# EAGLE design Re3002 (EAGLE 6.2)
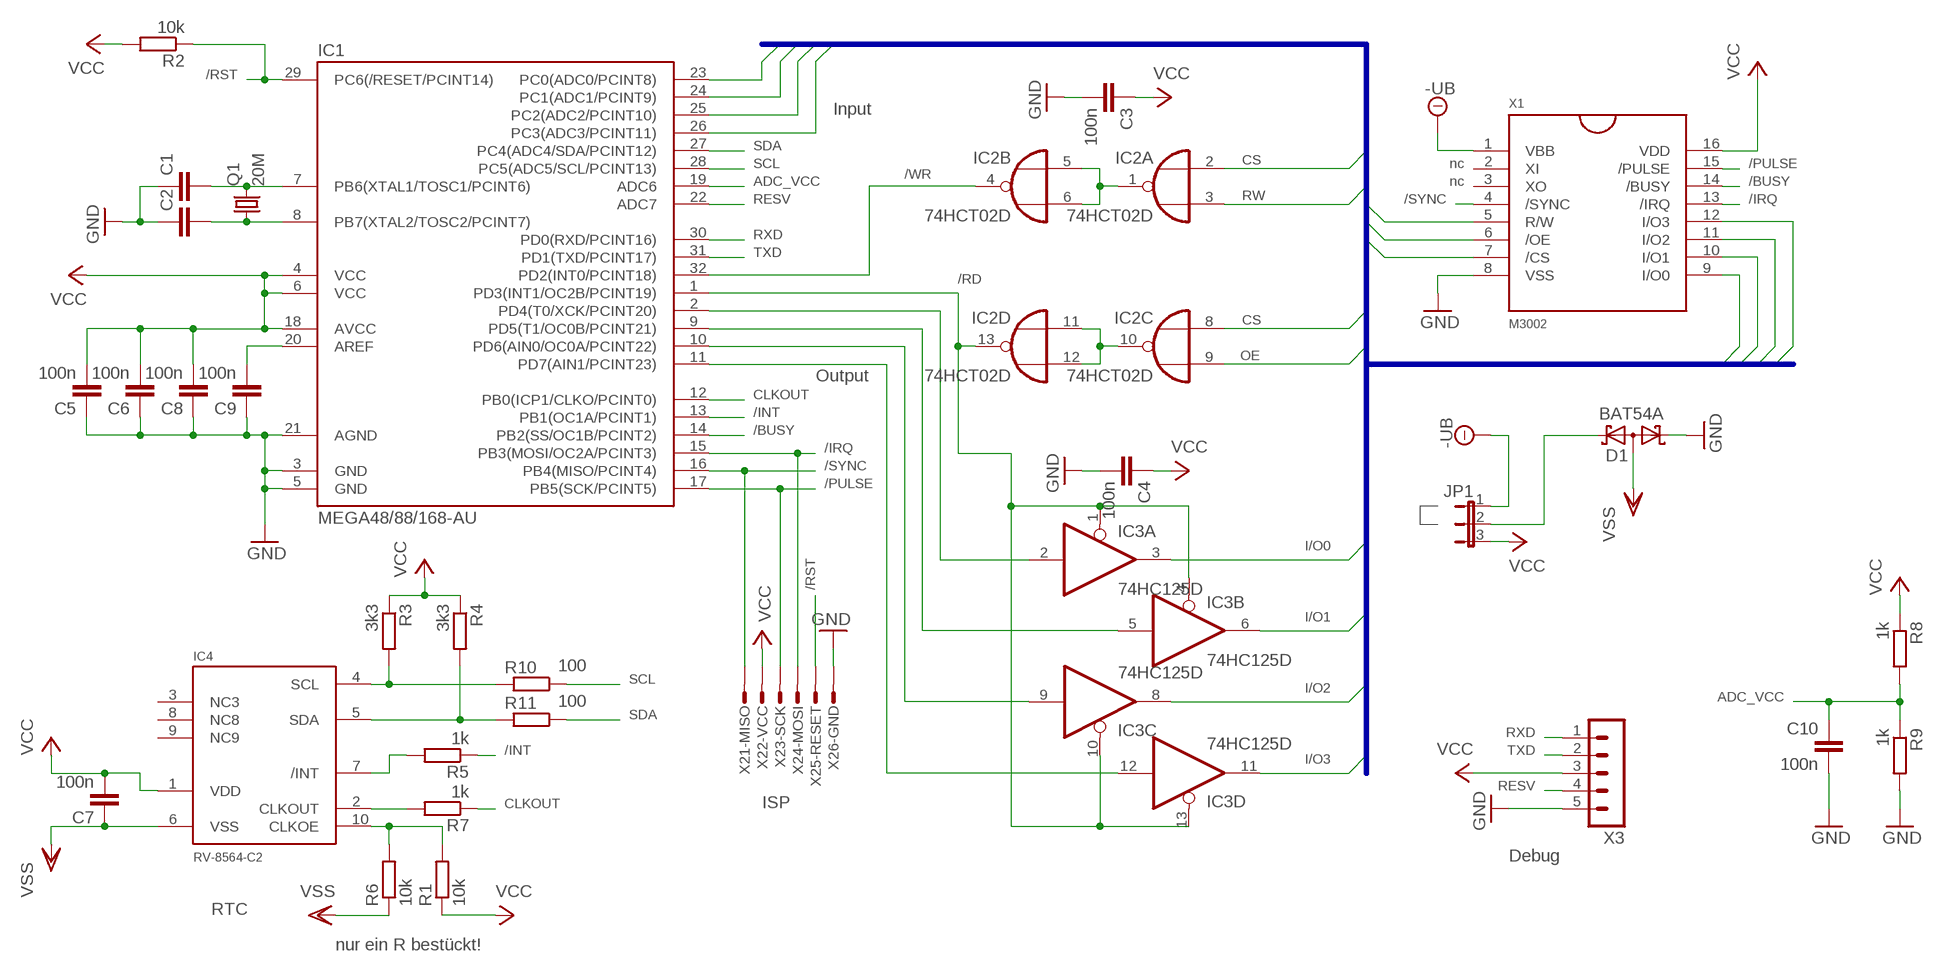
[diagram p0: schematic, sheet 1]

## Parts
C1  C-EUC0603  [C0603]
C2  C-EUC0603  [C0603]
C3  100n  C-EUC0603  [C0603]
C4  100n  C-EUC0603  [C0603]
C5  100n  C-EUC0603  [C0603]
C6  100n  C-EUC0603  [C0603]
C7  100n  C-EUC0603  [C0603]
C8  100n  C-EUC0603  [C0603]
C9  100n  C-EUC0603  [C0603]
C10  100n  C-EUC0603  [C0603]
D1  BAT54A  [SOT23]
IC1  MEGA48/88/168-AU  [TQFP32-08]
IC2  74HCT02D  [SO14]
IC3  74HC125D  [SO14]
IC4  RV-8564-C2  [RTC-MCS-50X32]
JP1  JP2E  [JP2]
Q1  20M  CRYSTALHC49S  [HC49/S]
R1  10k  R-EU_R0603  [R0603]
R2  10k  R-EU_R0603  [R0603]
R3  3k3  R-EU_R0603  [R0603]
R4  3k3  R-EU_R0603  [R0603]
R5  1k  R-EU_R0603  [R0603]
R6  10k  R-EU_R0603  [R0603]
R7  1k  R-EU_R0603  [R0603]
R8  1k  R-EU_R0603  [R0603]
R9  1k  R-EU_R0603  [R0603]
R10  100  R-EU_R0603  [R0603]
R11  100  R-EU_R0603  [R0603]
X1  M3002  [DIL-16]
X2  AVR-ISP_1X6  [1X6_ISP]
X3  MA05-1  [MA05-1]

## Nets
-UB: JP1.1 X1.1(VBB)
/BUSY: IC1.14(PB2(SS/OC1B/PCINT2)) X1.14(/BUSY)
/INT: IC1.13(PB1(OC1A/PCINT1)) R5.1
/IRQ: IC1.15(PB3(MOSI/OC2A/PCINT3)) X1.13(/IRQ) X2.4
/PULSE: IC1.17(PB5(SCK/PCINT5)) X1.15(/PULSE) X2.3
/RD: IC1.1(PD3(INT1/OC2B/PCINT19)) IC2.13(D:O) IC3.1(A:OE) IC3.4(B:OE) IC3.10(C:OE) IC3.13(D:OE)
/RST: IC1.29(PC6(/RESET/PCINT14)) R2.1 X2.5
/SYNC: IC1.16(PB4(MISO/PCINT4)) X1.4(/SYNC) X2.1
/WR: IC1.32(PD2(INT0/PCINT18)) IC2.4(B:O)
ADC_VCC: C10.1 IC1.19(ADC6) R8.2 R9.1
AREF: C9.2 IC1.20(AREF)
CLKOUT: IC1.12(PB0(ICP1/CLKO/PCINT0)) R7.1
CS: IC2.2(A:I0) IC2.8(C:I0) X1.7(/CS)
GND: C1.1 C2.1 C3.2 C4.2 C5.1 C6.1 C8.1 C9.1 C10.2 D1.1(K1) IC1.3(GND) IC1.5(GND) IC1.21(AGND) R9.2 X1.8(VSS) X2.6 X3.5
I/O0: IC1.23(PC0(ADC0/PCINT8)) IC3.3(A:O) X1.9(I/O0)
I/O1: IC1.24(PC1(ADC1/PCINT9)) IC3.6(B:O) X1.10(I/O1)
I/O2: IC1.25(PC2(ADC2/PCINT10)) IC3.8(C:O) X1.11(I/O2)
I/O3: IC1.26(PC3(ADC3/PCINT11)) IC3.11(D:O) X1.12(I/O3)
N$1: IC2.1(A:O) IC2.5(B:I0) IC2.6(B:I1)
N$2: IC2.10(C:O) IC2.11(D:I0) IC2.12(D:I1)
N$3: D1.2(K2) JP1.2
N$5: IC4.4(SCL) R3.2 R10.2
N$6: IC4.5(SDA) R4.2 R11.2
N$7: IC4.2(CLKOUT) R7.2
N$8: IC4.7(/INT) R5.2
N$9: C1.2 IC1.7(PB6(XTAL1/TOSC1/PCINT6)) Q1.2
N$10: C2.2 IC1.8(PB7(XTAL2/TOSC2/PCINT7)) Q1.1
N$12: IC4.10(CLKOE) R1.2 R6.2
OE: IC2.9(C:I1) X1.6(/OE)
OUT0: IC1.2(PD4(T0/XCK/PCINT20)) IC3.2(A:I)
OUT1: IC1.9(PD5(T1/OC0B/PCINT21)) IC3.5(B:I)
OUT2: IC1.10(PD6(AIN0/OC0A/PCINT22)) IC3.9(C:I)
OUT3: IC1.11(PD7(AIN1/PCINT23)) IC3.12(D:I)
RESV: IC1.22(ADC7) X3.4
RW: IC2.3(A:I1) X1.5(R/W)
RXD: IC1.30(PD0(RXD/PCINT16)) X3.1
SCL: IC1.28(PC5(ADC5/SCL/PCINT13)) R10.1
SDA: IC1.27(PC4(ADC4/SDA/PCINT12)) R11.1
TXD: IC1.31(PD1(TXD/PCINT17)) X3.2
VCC: C3.1 C4.1 C5.2 C6.2 C7.2 C8.2 IC1.4(VCC) IC1.6(VCC) IC1.18(AVCC) IC4.1(VDD) JP1.3 R1.1 R2.2 R3.1 R4.1 R8.1 X1.16(VDD) X2.2 X3.3
VSS: C7.1 D1.3(AA) IC4.6(VSS) R6.1
Unconnected: IC4.3(NC3) IC4.8(NC8) IC4.9(NC9) X1.2(XI) X1.3(XO)

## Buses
I/O[0..3],CS,RW,OE

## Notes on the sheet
- Input
- nc
- nc
- Output
- ISP
- Debug
- RTC
- nur ein R bestückt!

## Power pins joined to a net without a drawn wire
GND: IC2.7(P:GND) IC3.7(P:GND)
VCC: IC2.14(P:VCC) IC3.14(P:VCC)

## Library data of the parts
C1-C10 = rcl:C-EU: CAPACITOR, European symbol
D1 = diode:BAT54A: Schottky Diodes Source: Fairchild .. BAT54.pdf
IC1 = avr-7:MEGA48/88/168
IC2 = 74xx-eu:74*02: Quad 2-input NOR gate
IC3 = 74xx-eu:74*125: Quad bus BUFFER, 3-state
IC4 = misc:RV-8564-C2
JP1 = jumper:JP2E: JUMPER
Q1 = crystal:CRYSTAL: CRYSTAL; OC_FARNELL: 1667008; OC_NEWARK: unknown
R1-R11 = rcl:R-EU_: RESISTOR, European symbol
X1 = misc:M3002
X2 = 0_rr:AVR-ISP: MicroMaTch 6 7-215464-6 / 0-215464-6 Drawing Number C-215464 DDEController.pdf
X3 = con-lstb:MA05-1: PIN HEADER; OC_FARNELL: unknown; OC_NEWARK: unknown

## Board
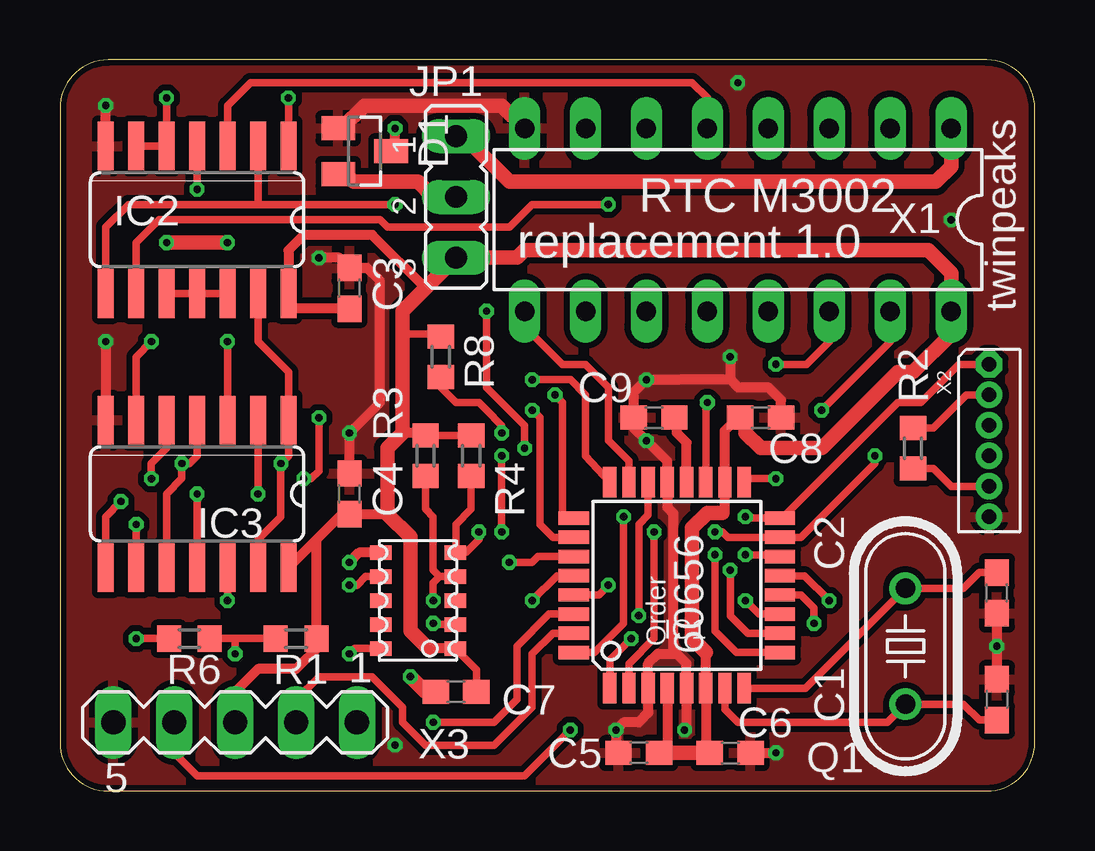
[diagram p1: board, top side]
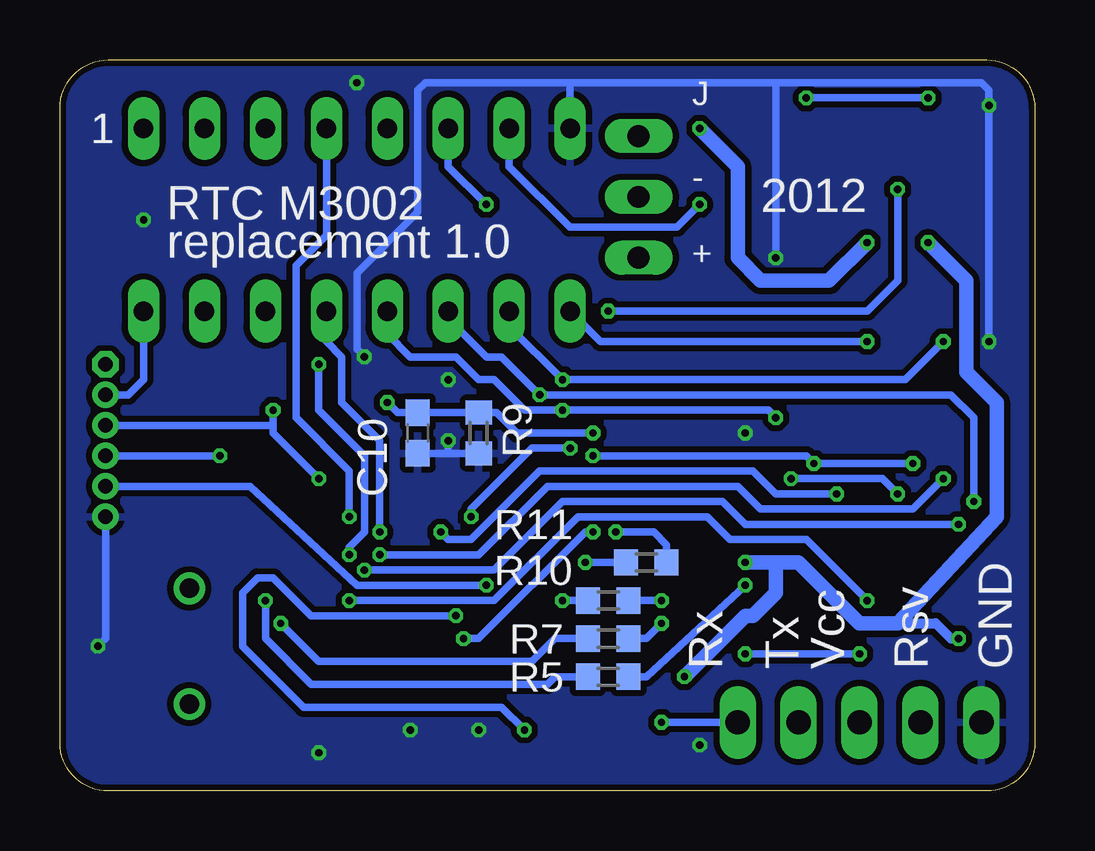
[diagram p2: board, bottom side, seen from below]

Size 40.63 x 30.47 mm. Coordinates in mm from the lower left corner, seen from the top.
Outline: 0,28.47 0,2 arc90 2,0 38.63,0 arc90 40.63,2 40.63,28.47 arc90 38.63,30.47 2,30.47 arc90 0,28.47
Copper layers (1*16): Top 0.035mm / dielectric 1.5mm / Bottom 0.035mm
Design rules: minimum track width 6mil, minimum drill 12mil, track to track 6mil, track to pad 6mil, pad to pad 6mil, via to via 6mil, smd to smd 0mil, copper to edge 10mil, drill to drill 10mil, minimum pad ring 10mil, minimum via ring 6mil, stop-mask expansion 2mil, vias tented up to drill 100mil, thermal gap 10mil

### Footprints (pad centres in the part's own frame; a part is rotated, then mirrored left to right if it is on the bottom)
C0603 = smd 1.1 x 1: 1 -0.85,0; 2 0.85,0
SOT23 = smd 1 x 1.4: 1 -0.95,-1.1; 2 0.95,-1.1; 3 0,1.1
TQFP32-08 = smd 1.27 x 0.559: 1 -4.293,2.8; 2 -4.293,2; 3 -4.293,1.2; 4 -4.293,0.4; 5 -4.293,-0.4; 6 -4.293,-1.2; 7 -4.293,-2; 8 -4.293,-2.8; 17 4.293,-2.8; 18 4.293,-2; 19 4.293,-1.2; 20 4.293,-0.4; 21 4.293,0.4; 22 4.293,1.2; 23 4.293,2; 24 4.293,2.8 | smd 0.559 x 1.27: 9 -2.8,-4.293; 10 -2,-4.293; 11 -1.2,-4.293; 12 -0.4,-4.293; 13 0.4,-4.293; 14 1.2,-4.293; 15 2,-4.293; 16 2.8,-4.293; 25 2.8,4.293; 26 2,4.293; 27 1.2,4.293; 28 0.4,4.293; 29 -0.4,4.293; 30 -1.2,4.293; 31 -2,4.293; 32 -2.8,4.293
SO14 = smd 0.66 x 2.032: 1 -3.81,-3.073; 2 -2.54,-3.073; 3 -1.27,-3.073; 4 0,-3.073; 5 1.27,-3.073; 6 2.54,-3.073; 7 3.81,-3.073; 8 3.81,3.073; 9 2.54,3.073; 10 1.27,3.073; 11 0,3.073; 12 -1.27,3.073; 13 -2.54,3.073; 14 -3.81,3.073
RTC-MCS-50X32 = smd 0.6 x 0.9: 1 -2,-1.55; 2 -1,-1.55; 3 0,-1.55; 4 1,-1.55; 5 2,-1.55; 6 2,1.55; 7 1,1.55; 8 0,1.55; 9 -1,1.55; 10 -2,1.55
JP2 = drill 0.914 long: 1 -2.54,0; 2 0,0; 3 2.54,0
HC49/S = drill 0.813: 1 -2.413,0; 2 2.413,0
R0603 = smd 1 x 1.1: 1 -0.85,0; 2 0.85,0
DIL-16 = drill 0.813 long: 1 -7.62,-3.81; 2 -5.08,-3.81; 3 -2.54,-3.81; 4 0,-3.81; 5 2.54,-3.81; 6 5.08,-3.81; 7 7.62,-3.81; 8 10.16,-3.81; 9 10.16,3.81; 10 7.62,3.81; 11 5.08,3.81; 12 2.54,3.81; 13 0,3.81; 14 -2.54,3.81; 15 -5.08,3.81; 16 -7.62,3.81
1X6_ISP = drill 0.6 pad 0.94 octagon: 1 0,0 | drill 0.6 pad 0.94: 2 1.27,0; 3 2.54,0; 4 3.81,0; 5 5.08,0; 6 6.35,0
MA05-1 = drill 1.016 long: 1 -5.08,0; 2 -2.54,0; 3 0,0; 4 2.54,0; 5 5.08,0

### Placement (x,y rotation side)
C1  39.05,3.81 270 top
C2  39.05,8.26 90 top
C3  12.06,20.95 90 top
C4  12.06,12.38 90 top
C5  24.13,1.59 0 top
C6  27.94,1.59 180 top
C7  16.51,4.13 0 top
C8  29.21,15.56 180 top
C9  24.77,15.56 0 top
C10  25.72,14.92 270 bottom
D1  12.7,26.67 270 top
IC1  25.72,8.57 90 top
IC2  5.71,23.81 180 top
IC3  5.71,12.38 180 top
IC4  14.92,7.94 90 top
JP1  16.51,24.77 270 top
Q1  35.24,6.03 270 top
R1  9.84,6.35 180 top
R2  35.56,14.29 90 top
R3  15.24,13.97 270 top
R4  17.14,13.97 270 top
R5  17.78,4.76 0 bottom
R6  5.4,6.35 0 top
R7  17.78,6.35 0 bottom
R8  15.88,18.1 270 top
R9  23.18,14.92 270 bottom
R10  17.78,7.94 0 bottom
R11  16.19,9.53 0 bottom
X1  29.53,23.81 180 top
X2  38.73,17.78 270 top
X3  7.3,2.86 180 top

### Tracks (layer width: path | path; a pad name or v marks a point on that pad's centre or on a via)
-UB
  Top 0.61: X1.1 37.15,26.04 36.51,25.4 21.27,25.4 21.59,25.4 18.73,25.4 16.83,27.3 JP1.1
/BUSY  (via drill 0.3)
  Top 0.305: X1.14 32.07,18.73 31.11,17.78 v29.84,17.78 | v28.57,9.84 29.94,9.84 IC1.14
  Bottom 0.305: v29.84,17.78 29.84,15.88 27.94,13.97 27.94,10.79 28.57,10.16 v28.57,9.84
/INT  (via drill 0.3)
  Top 0.305: IC1.13 31.03,8.97 v32.07,7.94
  Bottom 0.305: v32.07,7.94 32.07,6.35 30.16,4.45 20.32,4.45 20,4.76 R5.1
/IRQ  (via drill 0.3)
  Top 0.305: v33.97,13.97 33.97,13.65 30.89,10.57 IC1.15 27.84,10.57 27.62,10.79 v27.3,10.79
  Bottom 0.305: X1.13 29.53,18.73 28.89,18.1 28.89,16.19 27.3,14.61 v27.3,10.79 | v33.97,13.97 X2.4
/PULSE  (via drill 0.3)
  Top 0.305: X1.15 34.61,18.73 v31.75,15.88 | v29.84,13.02 28.67,13.02 IC1.17
  Bottom 0.305: v31.75,15.88 31.75,15.24 | X2.3 31.75,15.24 | 31.75,15.24 31.75,14.92 v29.84,13.02
/RD  (via drill 0.3)
  Top 0.305: IC2.13 8.26,18.73 9.53,17.46 IC3.1 9.53,13.97 v9.21,13.65 9.21,11.43 8.26,10.48 IC3.13 | IC3.4 5.71,13.97 5.4,13.65 v5.08,13.65 5.08,13.02 4.45,12.38 IC3.10 | v18.41,10.79 v18.41,13.97 | IC1.1 22.92,5.46 v23.81,6.35
  Bottom 0.305: v5.08,13.65 v9.21,13.65 9.53,13.97 v18.41,13.97 | v23.81,6.35 23.18,6.35 18.73,10.79 v18.41,10.79
/RST  (via drill 0.3)
  Top 0.305: IC1.29 22.46,8.17 v22.86,8.57 | R2.1 36.41,13.44 37.15,12.7 X2.5
  Bottom 0.305: v22.86,8.57 28.26,8.57 32.7,12.7 X2.5
/SYNC  (via drill 0.3)
  Top 0.305: v28.57,11.43 28.84,11.37 IC1.16 | X2.1 37.47,17.78 35.88,16.19 34.92,16.19 30.16,11.43
  Top 0.406: 30.16,11.43 30.01,11.43 IC1.16
  Bottom 0.305: X1.4 29.53,23.18 30.8,21.91 30.8,15.56 28.57,13.34 v28.57,11.43
/WR  (via drill 0.3)
  Top 0.305: IC2.4 v5.71,25.08 | v17.78,20 17.78,16.83 19.37,15.24 v19.37,14.29 | IC1.32 22.28,5.77 23.5,6.99 v23.5,11.43
  Bottom 0.305: v5.71,25.08 5.71,21.27 6.99,20 v17.78,20 | v23.5,11.43 23.5,11.75 20.95,14.29 v19.37,14.29
ADC_VCC  (via drill 0.3)
  Top 0.305: R8.2 15.88,16.83 16.51,16.19 17.46,16.19 17.78,15.88 18.41,15.24 v18.41,14.92 | IC1.19 26.92,16.12 v26.99,16.19
  Bottom 0.305: v18.41,14.92 21.59,14.92 22.44,15.77 R9.1 C10.1 26.57,15.77 v26.99,16.19
AREF
  Top 0.305: 25.72,15.46 C9.2
  Top 0.406: IC1.20 26.12,14.52 25.72,14.92 25.72,15.46
CLKOUT  (via drill 0.3)
  Top 0.305: IC1.12 30.88,8.17 31.43,7.62 v31.43,6.99
  Bottom 0.305: v31.43,6.99 29.84,5.4 20.95,5.4 20,6.35 R7.1
CS  (via drill 0.3)
  Top 0.305: IC2.2 8.26,24.45 | 8.26,24.45 2.86,24.45 1.91,23.5 IC2.8 | v13.97,24.45 8.26,24.45
  Bottom 0.305: X1.7 21.91,26.04 19.37,23.5 14.92,23.5 v13.97,24.45
GND  (via drill 0.3)
  Top 0.305: D1.1 11.74,27.62 | 23.18,1.69 C5.1 | 24.13,15.34 C9.1
  Top 0.406: IC2.7 v1.91,28.57 | v10.79,22.23 11.64,22.23 C3.2 12.8,21.8 13.34,21.27 13.34,16.19 v12.06,14.92 C4.2 | 25.56,5.71 25.56,11.59 25.32,11.83 IC1.21 25.32,13.73 v24.45,14.61 23.91,15.14 C9.1 23.91,16.61 v24.45,17.14 25.72,17.14 | 25.56,5.71 25.72,5.71 26.12,5.32 IC1.5 26.12,2.62 v26.04,2.54 | C2.1 v39.05,6.03 C1.1 | 25.56,5.71 24.92,5.71 24.52,5.31 IC1.3 24.52,3.25 24.13,2.86 23.5,2.86 v23.18,2.54 23.18,1.69 | v1.91,18.73 IC3.7 | v27.94,18.1 27.94,17.14 | C6.1 v29.84,1.59 | C8.1 30.06,16.3 29.53,16.83 28.26,16.83 27.94,17.14 | 27.94,17.14 25.82,17.14
  Top 0.61: 11.74,27.62 12.7,28.57 18.41,28.57 X1.8
  Bottom 0.305: X1.8 19.37,29.53 | 19.37,29.53 10.79,29.53 | 10.79,29.53 2.22,29.53 1.91,29.21 v1.91,28.57 v1.91,18.73 | v10.79,22.23 10.79,29.53 | X2.6 38.73,6.35 v39.05,6.03 | R9.2 24.45,14.07 | v27.94,18.1 28.26,18.41 28.26,21.59 25.72,24.13 25.72,29.21 25.4,29.53 19.37,29.53 | C10.2 24.45,14.07 | 24.45,14.07 v24.45,14.61
  other vias: 28.26,29.53 37.15,23.81 13.97,1.91
  pour Bottom (isolate 0.254): -0.95,31.43 41.59,31.43 41.59,-0.95 -0.95,-0.95
  pour Top (isolate 0.254): -0.32,30.8 40.96,30.8 40.96,-0.32 -0.32,-0.32
I/O0  (via drill 0.3)
  Top 0.305: v6.99,18.73 IC3.3 | X1.9 19.37,19.37 20.95,17.78 21.91,17.78 22.86,16.83 22.86,14.61 23.72,13.75 IC1.23
  Bottom 0.305: X1.9 18.1,18.73 v6.99,18.73
I/O1  (via drill 0.3)
  Top 0.305: v3.81,18.73 3.17,18.1 IC3.6 | IC1.24 21.91,13.97 21.91,16.51 21.27,17.14 v19.68,17.14
  Bottom 0.305: X1.10 21.91,19.37 v19.68,17.14 5.4,17.14 v3.81,18.73
I/O2  (via drill 0.3)
  Top 0.305: v2.54,12.06 1.91,11.43 IC3.8 | v20.64,16.51 20.95,16.19 20.95,11.43 21.01,11.37 IC1.25
  Bottom 0.305: X1.11 24.45,19.68 22.86,18.1 22.23,18.1 v20.64,16.51 3.49,16.51 2.54,15.56 v2.54,12.06
I/O3  (via drill 0.3)
  Top 0.305: v10.79,15.56 10.79,13.34 10.48,13.02 v10.16,13.02 | v5.71,12.38 IC3.11 | IC1.26 20.54,10.57 20,11.11 20,15.56 v19.68,15.88
  Bottom 0.305: X1.12 26.99,19.05 26.04,18.1 24.13,18.1 23.18,17.14 22.54,17.14 21.27,15.88 v19.68,15.88 11.11,15.88 v10.79,15.56 | v10.16,13.02 6.35,13.02 v5.71,12.38
N$1  (via drill 0.3)
  Top 0.305: IC2.6 IC2.5 v4.45,28.89 | v9.53,28.89 IC2.1
  Bottom 0.305: v4.45,28.89 v9.53,28.89
N$2
  Top 0.305: IC2.10 IC2.11 IC2.12
N$3
  Top 0.61: JP1.2 15.56,24.77 14.92,25.4 12.24,25.4 11.92,25.72 D1.2
N$5  (via drill 0.3)
  Top 0.305: R3.2 15.24,11.75 15.56,11.43 15.56,9.21 15.83,8.94 | 15.83,8.94 IC4.4 | v15.56,7.94 15.56,8.67 15.83,8.94
  Bottom 0.305: R10.2 v15.56,7.94
N$6  (via drill 0.3)
  Top 0.305: R4.2 17.14,11.75 16.51,11.11 16.51,9.97 IC4.5 16.92,9.94 17.46,10.48 v17.46,10.79
  Bottom 0.305: R11.2 15.34,10.26 15.88,10.79 v17.46,10.79
N$7  (via drill 0.3)
  Top 0.305: IC4.2 15.61,6.94 v15.56,6.99
  Bottom 0.305: v15.56,6.99 16.19,6.35 R7.2
N$8  (via drill 0.3)
  Top 0.305: IC4.7 12.75,8.94 12.38,8.57 v12.06,8.57
  Bottom 0.305: v12.06,8.57 16.19,4.76 R5.2
N$9
  Top 0.305: C1.2 38.31,2.96 37.66,3.62 Q1.2 34.48,2.86 28.26,2.86 27.72,3.4 IC1.7
N$10
  Top 0.305: C2.2 38.31,9.11 37.66,8.45 Q1.1 31.08,4.28 IC1.8
N$12  (via drill 0.3)
  Top 0.305: R6.2 7.3,6.35 | v7.3,5.71 7.3,6.35 | 7.3,6.35 R1.2 | IC4.10 12.29,5.94 v12.06,5.71
  Bottom 0.305: v12.06,5.71 v7.3,5.71
OE  (via drill 0.3)
  Top 0.305: v22.86,24.45 19.68,24.45 18.73,23.5 13.65,23.5 13.34,23.81 4.13,23.81 3.17,22.86 IC2.9
  Bottom 0.305: X1.6 24.45,26.04 v22.86,24.45
OUT0  (via drill 0.3)
  Top 0.305: IC3.2 v8.26,12.38 | IC1.2 23.72,5.3 24.77,6.35 v24.77,10.79
  Bottom 0.305: v24.77,10.79 24.45,10.48 23.5,10.48 20.64,13.34 11.75,13.34 10.79,12.38 v8.26,12.38
OUT1  (via drill 0.3)
  Top 0.305: IC3.5 4.45,14.29 3.81,13.65 v3.81,13.02 | v27.3,9.84 27.3,6.67 28.2,5.77 IC1.9
  Bottom 0.305: v3.81,13.02 5.08,11.75 11.43,11.75 12.38,12.7 20.32,12.7 23.18,9.84 v27.3,9.84
OUT2  (via drill 0.3)
  Top 0.305: IC3.9 v3.17,11.11 | IC1.10 28.67,6.57 27.94,7.3 v27.94,9.21
  Bottom 0.305: v3.17,11.11 12.06,11.11 13.02,12.06 19.68,12.06 22.54,9.21 v27.94,9.21
OUT3  (via drill 0.3)
  Top 0.305: IC3.12 v6.99,7.94 | IC1.11 29.14,7.37 v28.57,7.94
  Bottom 0.305: v6.99,7.94 9.53,10.48 12.7,10.48 13.65,11.43 19.05,11.43 22.54,7.94 v28.57,7.94
RESV  (via drill 0.3)
  Top 0.305: IC1.22 24.52,11.5 24.13,11.11 v24.13,7.3 | X3.4 4.76,1.59 5.71,0.64 19.37,0.64 v21.27,2.54
  Bottom 0.305: v24.13,7.3 30.16,7.3 31.75,8.89 32.38,8.89 33.02,8.26 33.02,6.03 30.48,3.49 22.23,3.49 v21.27,2.54
RW
  Top 0.305: IC2.3 6.99,28.57 7.94,29.53 26.35,29.53 26.99,28.89 X1.5
RXD  (via drill 0.3)
  Top 0.305: IC1.30 20.39,7.37 19.05,6.03 19.05,3.81 18.1,2.86 v15.56,2.86
  Bottom 0.305: v15.56,2.86 X3.1
SCL  (via drill 0.3)
  Top 0.305: v19.68,7.94 20.72,8.97 IC1.28
  Bottom 0.305: R10.1 v19.68,7.94
SDA  (via drill 0.3)
  Top 0.305: IC1.27 19.93,9.77 19.68,9.53 v18.73,9.53
  Bottom 0.305: R11.1 v18.73,9.53
TXD
  Top 0.305: IC1.31 20.54,6.57 19.68,5.71 19.68,3.49 18.1,1.91 15.24,1.91 14.29,2.86 14.29,3.49 13.02,4.76 10.79,4.76 9.84,3.81 X3.2
VCC
  Top 0.305: R2.2 36.41,15.14 37.78,16.51 X2.2 | R4.1 R3.1 | R8.1 15.88,19.05 14.29,19.05 | C6.2 26.92,1.76 26.75,1.59 | 25.32,1.93 C5.2 | C4.1 11.75,11.53 | R1.1 10.79,6.25 10.79,6.03 | 28.26,15.46 C8.2 28.57,15.34 | IC4.1 17.36,5.05 C7.2
  Top 0.406: X1.16 37.15,19.05 | 27.62,11.59 27.72,11.68 IC1.18 27.72,15.02 28.26,15.56 | 26.92,5.79 IC1.6 26.92,1.76 | IC1.4 25.32,1.93 | 13.65,11.53 C4.1 | 11.75,11.53 10.69,10.48 | 10.69,10.48 IC3.14 | IC4.1 15.34,5.94 | R1.1 10.69,10.48 | 10.79,6.03 9.84,5.08 8.26,5.08 7.3,4.13 X3.3 | R3.1 15.14,14.92 14.29,14.92 | 15.24,20.95 13.02,23.18 10.16,23.18 9.53,22.54 IC2.14 9.53,20.11 C3.1
  Top 0.61: X1.16 37.15,21.59 36.2,22.54 19.37,22.54 19.05,22.23 JP1.3 15.24,20.95 14.29,20 14.29,19.05 14.29,14.92 13.65,14.29 13.65,11.53 14.61,10.58 14.61,6.67 15.34,5.94 | 37.15,19.05 35.56,17.46 34.92,17.46 31.75,14.29 29.21,14.29 28.57,14.92 28.57,15.34 | 27.62,11.59 26.99,11.59 26.35,10.95 26.35,6.35 26.92,5.79 | 26.75,1.59 C5.2 | 28.26,15.56 28.26,15.46
  Bottom 0.305: X2.2 37.78,16.51 37.15,17.14 X1.16
VSS  (via drill 0.3)
  Top 0.305: R6.1 v3.17,6.35 | C7.1 15.24,4.13
  Top 0.406: D1.3 13.97,26.5 v13.97,27.62 | 13.43,9.94 IC4.6 12.48,9.94 v12.06,9.53
  Top 0.61: v6.99,22.86 v4.45,22.86 | 15.24,4.13 v14.61,4.76
  Bottom 0.406: 5.71,6.99 4.13,6.99 3.49,6.35 v3.17,6.35
  Bottom 0.61: v13.97,27.62 12.38,26.04 12.38,22.23 11.43,21.27 8.57,21.27 v6.99,22.86 | v4.45,22.86 2.86,21.27 2.86,17.46 1.59,16.19 1.59,11.43 5.71,6.99 7.3,6.99 9.84,9.53 10.79,9.53 | v12.06,9.53 10.79,9.53 | v14.61,4.76 12.06,7.3 11.75,7.3 10.79,8.26 10.79,9.53

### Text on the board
tPlace: RTC M3002 | replacement 1.0 | twinpeaks | Order | 60656
bPlace: J | 1 | - | 2012 | RTC M3002 | + | replacement 1.0 | GND | Rsv | Vcc | Tx | Rx
bStop: twinpeaks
